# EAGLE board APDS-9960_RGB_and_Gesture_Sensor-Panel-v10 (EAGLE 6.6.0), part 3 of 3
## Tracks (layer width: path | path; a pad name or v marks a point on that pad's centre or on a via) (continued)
VCC27  (via drill 0.38) (continued)
  Top 0.762: 102.62,80.75 v102.62,82.04 v102.62,83.06
  Bottom 0.305: v115.06,82.68 115.06,81.15 v114.05,80.14
  Bottom 0.762: v102.62,83.06 v102.62,82.04 102.62,81.28 107.7,76.2 JP28.3
VCC28  (via drill 0.38)
  Top 0.305: SJ57.2 v19.56,100.97 | v20.57,103.5 R113.2 19.14,104.31 18.8,104.65 18.29,104.65 16,106.93 16,107.95 14.99,108.97 13.97,108.97 12.7,107.7 12.7,106.86
  Top 0.559: 9.61,101.81 9.18,101.38 SJ58.2 8.13,101.58 | R115.2 9.61,101.81 | 9.61,101.81 9.61,102.58 9.82,102.78 C86.1 9.82,104.56 12.12,106.86 12.7,106.86 U29.8
  Top 0.762: 8.13,101.58 v8.13,102.87 v8.13,103.89
  Bottom 0.305: v20.57,103.5 20.57,101.98 v19.56,100.97
  Bottom 0.762: v8.13,103.89 v8.13,102.87 8.13,102.11 13.21,97.03 JP29.3
VCC29  (via drill 0.38)
  Top 0.305: SJ59.2 v35.31,100.97 | v36.32,103.5 R117.2 34.89,104.31 34.54,104.65 34.04,104.65 31.75,106.93 31.75,107.95 30.73,108.97 29.72,108.97 28.45,107.7 28.45,106.86
  Top 0.559: 25.36,101.81 24.92,101.38 SJ60.2 23.88,101.58 | R119.2 25.36,101.81 | 25.36,101.81 25.36,102.58 25.57,102.78 C89.1 25.57,104.56 27.87,106.86 28.45,106.86 U30.8
  Top 0.762: 23.88,101.58 v23.88,102.87 v23.88,103.89
  Bottom 0.305: v36.32,103.5 36.32,101.98 v35.31,100.97
  Bottom 0.762: v23.88,103.89 v23.88,102.87 23.88,102.11 28.96,97.03 JP30.3
VCC30  (via drill 0.38)
  Top 0.305: SJ61.2 v51.05,100.97 | v52.07,103.5 R121.2 50.63,104.31 50.29,104.65 49.78,104.65 47.5,106.93 47.5,107.95 46.48,108.97 45.47,108.97 44.2,107.7 44.2,106.86
  Top 0.559: 41.11,101.81 40.67,101.38 SJ62.2 39.62,101.58 | R123.2 41.11,101.81 | 41.11,101.81 41.11,102.58 41.31,102.78 C92.1 41.31,104.56 43.62,106.86 44.2,106.86 U31.8
  Top 0.762: 39.62,101.58 v39.62,102.87 v39.62,103.89
  Bottom 0.305: v52.07,103.5 52.07,101.98 v51.05,100.97
  Bottom 0.762: v39.62,103.89 v39.62,102.87 39.62,102.11 44.7,97.03 JP31.3
VCC31  (via drill 0.38)
  Top 0.305: SJ63.2 v66.8,100.97 | v67.82,103.5 R125.2 66.38,104.31 66.04,104.65 65.53,104.65 63.25,106.93 63.25,107.95 62.23,108.97 61.21,108.97 59.94,107.7 59.94,106.86
  Top 0.559: 56.86,101.81 56.42,101.38 SJ64.2 55.37,101.58 | R127.2 56.86,101.81 | 56.86,101.81 56.86,102.58 57.06,102.78 C95.1 57.06,104.56 59.37,106.86 59.94,106.86 U32.8
  Top 0.762: 55.37,101.58 v55.37,102.87 v55.37,103.89
  Bottom 0.305: v67.82,103.5 67.82,101.98 v66.8,100.97
  Bottom 0.762: v55.37,103.89 v55.37,102.87 55.37,102.11 60.45,97.03 JP32.3
VCC32  (via drill 0.38)
  Top 0.305: SJ65.2 v82.55,100.97 | v83.57,103.5 R129.2 82.13,104.31 81.79,104.65 81.28,104.65 78.99,106.93 78.99,107.95 77.98,108.97 76.96,108.97 75.69,107.7 75.69,106.86
  Top 0.559: 72.61,101.81 72.17,101.38 SJ66.2 71.12,101.58 | R131.2 72.61,101.81 | 72.61,101.81 72.61,102.58 72.81,102.78 C98.1 72.81,104.56 75.11,106.86 75.69,106.86 U33.8
  Top 0.762: 71.12,101.58 v71.12,102.87 v71.12,103.89
  Bottom 0.305: v83.57,103.5 83.57,101.98 v82.55,100.97
  Bottom 0.762: v71.12,103.89 v71.12,102.87 71.12,102.11 76.2,97.03 JP33.3
VCC33  (via drill 0.38)
  Top 0.305: SJ67.2 v98.3,100.97 | v99.31,103.5 R133.2 97.88,104.31 97.54,104.65 97.03,104.65 94.74,106.93 94.74,107.95 93.73,108.97 92.71,108.97 91.44,107.7 91.44,106.86
  Top 0.559: 88.35,101.81 87.92,101.38 SJ68.2 86.87,101.58 | R135.2 88.35,101.81 | 88.35,101.81 88.35,102.58 88.56,102.78 C101.1 88.56,104.56 90.86,106.86 91.44,106.86 U34.8
  Top 0.762: 86.87,101.58 v86.87,102.87 v86.87,103.89
  Bottom 0.305: v99.31,103.5 99.31,101.98 v98.3,100.97
  Bottom 0.762: v86.87,103.89 v86.87,102.87 86.87,102.11 91.95,97.03 JP34.3
VCC34  (via drill 0.38)
  Top 0.305: SJ69.2 v114.05,100.97 | v115.06,103.5 R137.2 113.63,104.31 113.28,104.65 112.78,104.65 110.49,106.93 110.49,107.95 109.47,108.97 108.46,108.97 107.19,107.7 107.19,106.86
  Top 0.559: 104.1,101.81 103.66,101.38 SJ70.2 102.62,101.58 | R139.2 104.1,101.81 | 104.1,101.81 104.1,102.58 104.31,102.78 C104.1 104.31,104.56 106.61,106.86 107.19,106.86 U35.8
  Top 0.762: 102.62,101.58 v102.62,102.87 v102.62,103.89
  Bottom 0.305: v115.06,103.5 115.06,101.98 v114.05,100.97
  Bottom 0.762: v102.62,103.89 v102.62,102.87 102.62,102.11 107.7,97.03 JP35.3
VL
  Top 0.559: SJ2.1 9.18,17.24 9.61,16.8 R4.1 11.47,16.8 11.94,17.27 11.94,18.03 12.41,18.5 C2.1 13.78,19.07 U1.5
  Top 0.762: R4.1 10.67,15.75 11.31,15.11 C1.A 9.14,13.21 8.13,12.19 JP1.1
VL1
  Top 0.559: SJ4.1 24.92,17.24 25.36,16.8 R7.1 27.22,16.8 27.69,17.27 27.69,18.03 28.16,18.5 C4.1 29.53,19.07 U2.5
  Top 0.762: R7.1 26.42,15.75 27.06,15.11 C6.A 24.89,13.21 23.88,12.19 JP2.1
VL2
  Top 0.559: SJ6.1 40.67,17.24 41.11,16.8 R11.1 42.97,16.8 43.43,17.27 43.43,18.03 43.9,18.5 C7.1 45.27,19.07 U3.5
  Top 0.762: R11.1 42.16,15.75 42.8,15.11 C9.A 40.64,13.21 39.62,12.19 JP3.1
VL3
  Top 0.559: SJ8.1 56.42,17.24 56.86,16.8 R15.1 58.71,16.8 59.18,17.27 59.18,18.03 59.65,18.5 C10.1 61.02,19.07 U4.5
  Top 0.762: R15.1 57.91,15.75 58.55,15.11 C12.A 56.39,13.21 55.37,12.19 JP4.1
VL4
  Top 0.559: SJ10.1 72.17,17.24 72.61,16.8 R19.1 74.46,16.8 74.93,17.27 74.93,18.03 75.4,18.5 C13.1 76.77,19.07 U5.5
  Top 0.762: R19.1 73.66,15.75 74.3,15.11 C15.A 72.14,13.21 71.12,12.19 JP5.1
VL5
  Top 0.559: SJ12.1 87.92,17.24 88.35,16.8 R23.1 90.21,16.8 90.68,17.27 90.68,18.03 91.15,18.5 C16.1 92.52,19.07 U6.5
  Top 0.762: R23.1 89.41,15.75 90.05,15.11 C18.A 87.88,13.21 86.87,12.19 JP6.1
VL6
  Top 0.559: SJ14.1 103.66,17.24 104.1,16.8 R27.1 105.96,16.8 106.43,17.27 106.43,18.03 106.89,18.5 C19.1 108.27,19.07 U7.5
  Top 0.762: R27.1 105.16,15.75 105.8,15.11 C21.A 103.63,13.21 102.62,12.19 JP7.1
VL7
  Top 0.559: SJ16.1 9.18,38.07 9.61,37.63 R31.1 11.47,37.63 11.94,38.1 11.94,38.86 12.41,39.33 C22.1 13.78,39.9 U8.5
  Top 0.762: R31.1 10.67,36.58 11.31,35.94 C24.A 9.14,34.04 8.13,33.02 JP8.1
VL8
  Top 0.559: SJ18.1 24.92,38.07 25.36,37.63 R35.1 27.22,37.63 27.69,38.1 27.69,38.86 28.16,39.33 C25.1 29.53,39.9 U9.5
  Top 0.762: R35.1 26.42,36.58 27.06,35.94 C27.A 24.89,34.04 23.88,33.02 JP9.1
VL9
  Top 0.559: SJ20.1 40.67,38.07 41.11,37.63 R39.1 42.97,37.63 43.43,38.1 43.43,38.86 43.9,39.33 C28.1 45.27,39.9 U10.5
  Top 0.762: R39.1 42.16,36.58 42.8,35.94 C30.A 40.64,34.04 39.62,33.02 JP10.1
VL10
  Top 0.559: SJ22.1 56.42,38.07 56.86,37.63 R43.1 58.71,37.63 59.18,38.1 59.18,38.86 59.65,39.33 C31.1 61.02,39.9 U11.5
  Top 0.762: R43.1 57.91,36.58 58.55,35.94 C33.A 56.39,34.04 55.37,33.02 JP11.1
VL11
  Top 0.559: SJ24.1 72.17,38.07 72.61,37.63 R47.1 74.46,37.63 74.93,38.1 74.93,38.86 75.4,39.33 C34.1 76.77,39.9 U12.5
  Top 0.762: R47.1 73.66,36.58 74.3,35.94 C36.A 72.14,34.04 71.12,33.02 JP12.1
VL12
  Top 0.559: SJ26.1 87.92,38.07 88.35,37.63 R51.1 90.21,37.63 90.68,38.1 90.68,38.86 91.15,39.33 C37.1 92.52,39.9 U13.5
  Top 0.762: R51.1 89.41,36.58 90.05,35.94 C39.A 87.88,34.04 86.87,33.02 JP13.1
VL13
  Top 0.559: SJ28.1 103.66,38.07 104.1,37.63 R55.1 105.96,37.63 106.43,38.1 106.43,38.86 106.89,39.33 C40.1 108.27,39.9 U14.5
  Top 0.762: R55.1 105.16,36.58 105.8,35.94 C42.A 103.63,34.04 102.62,33.02 JP14.1
VL14
  Top 0.559: SJ30.1 9.18,58.9 9.61,58.46 R59.1 11.47,58.46 11.94,58.93 11.94,59.69 12.41,60.16 C43.1 13.78,60.73 U15.5
  Top 0.762: R59.1 10.67,57.4 11.31,56.76 C45.A 9.14,54.86 8.13,53.85 JP15.1
VL15
  Top 0.559: SJ32.1 24.92,58.9 25.36,58.46 R63.1 27.22,58.46 27.69,58.93 27.69,59.69 28.16,60.16 C46.1 29.53,60.73 U16.5
  Top 0.762: R63.1 26.42,57.4 27.06,56.76 C48.A 24.89,54.86 23.88,53.85 JP16.1
VL16
  Top 0.559: SJ34.1 40.67,58.9 41.11,58.46 R67.1 42.97,58.46 43.43,58.93 43.43,59.69 43.9,60.16 C49.1 45.27,60.73 U17.5
  Top 0.762: R67.1 42.16,57.4 42.8,56.76 C51.A 40.64,54.86 39.62,53.85 JP17.1
VL17
  Top 0.559: SJ36.1 56.42,58.9 56.86,58.46 R71.1 58.71,58.46 59.18,58.93 59.18,59.69 59.65,60.16 C52.1 61.02,60.73 U18.5
  Top 0.762: R71.1 57.91,57.4 58.55,56.76 C54.A 56.39,54.86 55.37,53.85 JP18.1
VL18
  Top 0.559: SJ38.1 72.17,58.9 72.61,58.46 R75.1 74.46,58.46 74.93,58.93 74.93,59.69 75.4,60.16 C55.1 76.77,60.73 U19.5
  Top 0.762: R75.1 73.66,57.4 74.3,56.76 C57.A 72.14,54.86 71.12,53.85 JP19.1
VL19
  Top 0.559: SJ40.1 87.92,58.9 88.35,58.46 R79.1 90.21,58.46 90.68,58.93 90.68,59.69 91.15,60.16 C58.1 92.52,60.73 U20.5
  Top 0.762: R79.1 89.41,57.4 90.05,56.76 C60.A 87.88,54.86 86.87,53.85 JP20.1
VL20
  Top 0.559: SJ42.1 103.66,58.9 104.1,58.46 R83.1 105.96,58.46 106.43,58.93 106.43,59.69 106.89,60.16 C61.1 108.27,60.73 U21.5
  Top 0.762: R83.1 105.16,57.4 105.8,56.76 C63.A 103.63,54.86 102.62,53.85 JP21.1
VL21
  Top 0.559: SJ44.1 9.18,79.72 9.61,79.29 R87.1 11.47,79.29 11.94,79.76 11.94,80.52 12.41,80.99 C64.1 13.78,81.56 U22.5
  Top 0.762: R87.1 10.67,78.23 11.31,77.59 C66.A 9.14,75.69 8.13,74.68 JP22.1
VL22
  Top 0.559: SJ46.1 24.92,79.72 25.36,79.29 R91.1 27.22,79.29 27.69,79.76 27.69,80.52 28.16,80.99 C67.1 29.53,81.56 U23.5
  Top 0.762: R91.1 26.42,78.23 27.06,77.59 C69.A 24.89,75.69 23.88,74.68 JP23.1
VL23
  Top 0.559: SJ48.1 40.67,79.72 41.11,79.29 R95.1 42.97,79.29 43.43,79.76 43.43,80.52 43.9,80.99 C70.1 45.27,81.56 U24.5
  Top 0.762: R95.1 42.16,78.23 42.8,77.59 C72.A 40.64,75.69 39.62,74.68 JP24.1
VL24
  Top 0.559: SJ50.1 56.42,79.72 56.86,79.29 R99.1 58.71,79.29 59.18,79.76 59.18,80.52 59.65,80.99 C73.1 61.02,81.56 U25.5
  Top 0.762: R99.1 57.91,78.23 58.55,77.59 C75.A 56.39,75.69 55.37,74.68 JP25.1
VL25
  Top 0.559: SJ52.1 72.17,79.72 72.61,79.29 R103.1 74.46,79.29 74.93,79.76 74.93,80.52 75.4,80.99 C76.1 76.77,81.56 U26.5
  Top 0.762: R103.1 73.66,78.23 74.3,77.59 C78.A 72.14,75.69 71.12,74.68 JP26.1
VL26
  Top 0.559: SJ54.1 87.92,79.72 88.35,79.29 R107.1 90.21,79.29 90.68,79.76 90.68,80.52 91.15,80.99 C79.1 92.52,81.56 U27.5
  Top 0.762: R107.1 89.41,78.23 90.05,77.59 C81.A 87.88,75.69 86.87,74.68 JP27.1
VL27
  Top 0.559: SJ56.1 103.66,79.72 104.1,79.29 R111.1 105.96,79.29 106.43,79.76 106.43,80.52 106.89,80.99 C82.1 108.27,81.56 U28.5
  Top 0.762: R111.1 105.16,78.23 105.8,77.59 C84.A 103.63,75.69 102.62,74.68 JP28.1
VL28
  Top 0.559: SJ58.1 9.18,100.55 9.61,100.11 R115.1 11.47,100.11 11.94,100.58 11.94,101.35 12.41,101.81 C85.1 13.78,102.39 U29.5
  Top 0.762: R115.1 10.67,99.06 11.31,98.42 C87.A 9.14,96.52 8.13,95.5 JP29.1
VL29
  Top 0.559: SJ60.1 24.92,100.55 25.36,100.11 R119.1 27.22,100.11 27.69,100.58 27.69,101.35 28.16,101.81 C88.1 29.53,102.39 U30.5
  Top 0.762: R119.1 26.42,99.06 27.06,98.42 C90.A 24.89,96.52 23.88,95.5 JP30.1
VL30
  Top 0.559: SJ62.1 40.67,100.55 41.11,100.11 R123.1 42.97,100.11 43.43,100.58 43.43,101.35 43.9,101.81 C91.1 45.27,102.39 U31.5
  Top 0.762: R123.1 42.16,99.06 42.8,98.42 C93.A 40.64,96.52 39.62,95.5 JP31.1
VL31
  Top 0.559: SJ64.1 56.42,100.55 56.86,100.11 R127.1 58.71,100.11 59.18,100.58 59.18,101.35 59.65,101.81 C94.1 61.02,102.39 U32.5
  Top 0.762: R127.1 57.91,99.06 58.55,98.42 C96.A 56.39,96.52 55.37,95.5 JP32.1
VL32
  Top 0.559: SJ66.1 72.17,100.55 72.61,100.11 R131.1 74.46,100.11 74.93,100.58 74.93,101.35 75.4,101.81 C97.1 76.77,102.39 U33.5
  Top 0.762: R131.1 73.66,99.06 74.3,98.42 C99.A 72.14,96.52 71.12,95.5 JP33.1
VL33
  Top 0.559: SJ68.1 87.92,100.55 88.35,100.11 R135.1 90.21,100.11 90.68,100.58 90.68,101.35 91.15,101.81 C100.1 92.52,102.39 U34.5
  Top 0.762: R135.1 89.41,99.06 90.05,98.42 C102.A 87.88,96.52 86.87,95.5 JP34.1
VL34
  Top 0.559: SJ70.1 103.66,100.55 104.1,100.11 R139.1 105.96,100.11 106.43,100.58 106.43,101.35 106.89,101.81 C103.1 108.27,102.39 U35.5
  Top 0.762: R139.1 105.16,99.06 105.8,98.42 C105.A 103.63,96.52 102.62,95.5 JP35.1

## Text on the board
Bottom: v10 | v10 | v10 | v10 | v10 | v10 | v10 | v10 | v10 | v10 | v10 | v10 | v10 | v10 | v10 | v10 | v10 | v10 | v10 | v10 | v10 | v10 | v10 | v10 | v10 | v10 | v10 | v10 | v10 | v10 | v10 | v10 | v10 | v10 | v10
tPlace: PS | PS | PS | PS | PS | PS | PS | I2C | PU | I2C | PU | I2C | PU | I2C | PU | I2C | PU | I2C | PU | I2C | PU | VL | GND | VCC | SDA | SCL | INT | VL | GND | VCC | SDA | SCL | INT | VL | GND | VCC | SDA | SCL | INT | VL | GND | VCC | SDA | SCL | INT | VL | GND | VCC | SDA | SCL | INT | VL | GND | VCC | SDA | SCL | INT | VL | GND | VCC | SDA | SCL | INT | PS | PS | PS | PS | PS | PS | PS | I2C | PU | I2C | PU | I2C | PU | I2C | PU | I2C | PU | I2C | PU | I2C | PU | VL | GND | VCC | SDA | SCL | INT | VL | GND | VCC | SDA | SCL | INT | VL | GND | VCC | SDA | SCL | INT | VL | GND | VCC | SDA | SCL | INT | VL | GND | VCC | SDA | SCL | INT | VL | GND | VCC | SDA | SCL | INT | VL | GND | VCC | SDA | SCL | INT | PS | PS | PS | PS | PS | PS | PS | I2C | PU | I2C | PU | I2C | PU | I2C | PU | I2C | PU | I2C | PU | I2C | PU | VL | GND | VCC | SDA | SCL | INT | VL | GND | VCC | SDA | SCL | INT | VL | GND | VCC | SDA | SCL | INT | VL | GND | VCC | SDA | SCL | INT | VL | GND | VCC | SDA | SCL | INT | VL | GND | VCC | SDA | SCL | INT | VL | GND | VCC | SDA | SCL | INT | PS | PS | PS | PS | PS | PS | PS | I2C | PU | I2C | PU | I2C | PU | I2C | PU | I2C | PU | I2C | PU | I2C | PU | VL | GND | VCC | SDA | SCL | INT | VL | GND | VCC | SDA | SCL | INT | VL | GND | VCC | SDA | SCL | INT | VL | GND | VCC | SDA | SCL | INT | VL | GND | VCC | SDA | SCL | INT | VL | GND | VCC | SDA | SCL | INT | VL | GND | VCC | SDA | SCL | INT | PS | PS | PS | PS | PS | PS | PS | I2C | PU | I2C | PU | I2C | PU | I2C | PU | I2C | PU | I2C | PU | I2C | PU | VL | GND | VCC | SDA | SCL | INT | VL | GND | VCC | SDA | SCL | INT | VL | GND | VCC | SDA | SCL | INT | VL | GND | VCC | SDA | SCL | INT | VL | GND | VCC | SDA | SCL | INT | VL | GND | VCC | SDA | SCL | INT | VL | GND | VCC | SDA | SCL | INT
bPlace: APDS-9960 | APDS-9960 | APDS-9960 | APDS-9960 | APDS-9960 | APDS-9960 | APDS-9960 | I2C: 0x39 | RGB/Gesture | I2C: 0x39 | RGB/Gesture | I2C: 0x39 | RGB/Gesture | I2C: 0x39 | RGB/Gesture | I2C: 0x39 | RGB/Gesture | I2C: 0x39 | RGB/Gesture | I2C: 0x39 | RGB/Gesture | VL | GND | VCC | SDA | SCL | INT | VL | GND | VCC | SDA | SCL | INT | VL | GND | VCC | SDA | SCL | INT | VL | GND | VCC | SDA | SCL | INT | VL | GND | VCC | SDA | SCL | INT | VL | GND | VCC | SDA | SCL | INT | VL | GND | VCC | SDA | SCL | INT | APDS-9960 | APDS-9960 | APDS-9960 | APDS-9960 | APDS-9960 | APDS-9960 | APDS-9960 | I2C: 0x39 | RGB/Gesture | I2C: 0x39 | RGB/Gesture | I2C: 0x39 | RGB/Gesture | I2C: 0x39 | RGB/Gesture | I2C: 0x39 | RGB/Gesture | I2C: 0x39 | RGB/Gesture | I2C: 0x39 | RGB/Gesture | VL | GND | VCC | SDA | SCL | INT | VL | GND | VCC | SDA | SCL | INT | VL | GND | VCC | SDA | SCL | INT | VL | GND | VCC | SDA | SCL | INT | VL | GND | VCC | SDA | SCL | INT | VL | GND | VCC | SDA | SCL | INT | VL | GND | VCC | SDA | SCL | INT | APDS-9960 | APDS-9960 | APDS-9960 | APDS-9960 | APDS-9960 | APDS-9960 | APDS-9960 | I2C: 0x39 | RGB/Gesture | I2C: 0x39 | RGB/Gesture | I2C: 0x39 | RGB/Gesture | I2C: 0x39 | RGB/Gesture | I2C: 0x39 | RGB/Gesture | I2C: 0x39 | RGB/Gesture | I2C: 0x39 | RGB/Gesture | VL | GND | VCC | SDA | SCL | INT | VL | GND | VCC | SDA | SCL | INT | VL | GND | VCC | SDA | SCL | INT | VL | GND | VCC | SDA | SCL | INT | VL | GND | VCC | SDA | SCL | INT | VL | GND | VCC | SDA | SCL | INT | VL | GND | VCC | SDA | SCL | INT | APDS-9960 | APDS-9960 | APDS-9960 | APDS-9960 | APDS-9960 | APDS-9960 | APDS-9960 | I2C: 0x39 | RGB/Gesture | I2C: 0x39 | RGB/Gesture | I2C: 0x39 | RGB/Gesture | I2C: 0x39 | RGB/Gesture | I2C: 0x39 | RGB/Gesture | I2C: 0x39 | RGB/Gesture | I2C: 0x39 | RGB/Gesture | VL | GND | VCC | SDA | SCL | INT | VL | GND | VCC | SDA | SCL | INT | VL | GND | VCC | SDA | SCL | INT | VL | GND | VCC | SDA | SCL | INT | VL | GND | VCC | SDA | SCL | INT | VL | GND | VCC | SDA | SCL | INT | VL | GND | VCC | SDA | SCL | INT | APDS-9960 | APDS-9960 | APDS-9960 | APDS-9960 | APDS-9960 | APDS-9960 | APDS-9960 | I2C: 0x39 | RGB/Gesture | I2C: 0x39 | RGB/Gesture | I2C: 0x39 | RGB/Gesture | I2C: 0x39 | RGB/Gesture | I2C: 0x39 | RGB/Gesture | I2C: 0x39 | RGB/Gesture | I2C: 0x39 | RGB/Gesture | VL | GND | VCC | SDA | SCL | INT | VL | GND | VCC | SDA | SCL | INT | VL | GND | VCC | SDA | SCL | INT | VL | GND | VCC | SDA | SCL | INT | VL | GND | VCC | SDA | SCL | INT | VL | GND | VCC | SDA | SCL | INT | VL | GND | VCC | SDA | SCL | INT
